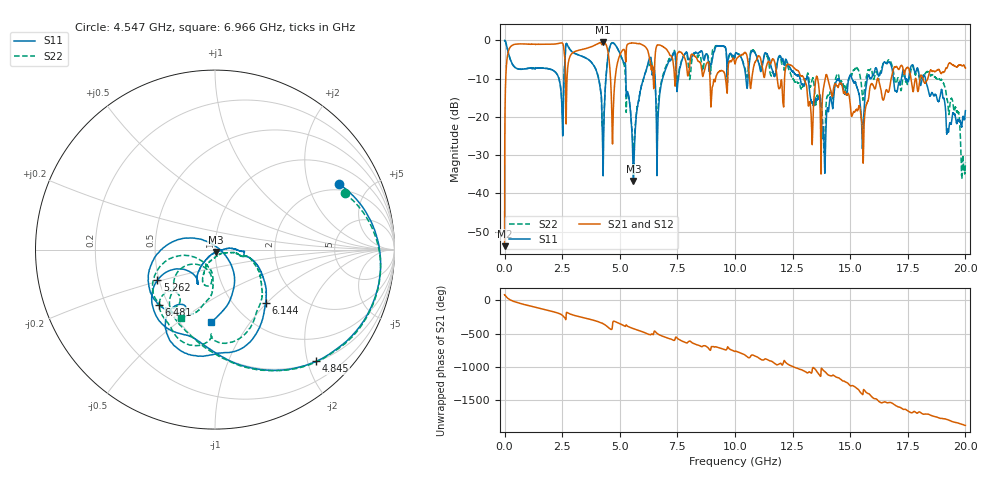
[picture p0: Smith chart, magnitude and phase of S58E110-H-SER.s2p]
!{S58E110}
!Johanson Technology Inc.
!www.johansontechnology.com
!Test Board Conditions:
!Substrate Type  RO4350B
!Substrate Thickness  60 mil
!Substrate Dk  3.66
!TL Type: GCPW
!TL Trace Width  115 mil
!TL Gap  52 mil
!Electrode orientation  Horizontal
!DUT TOPOLOGY	SERIES
!Mounting Pad LxW  55x428 mil
! Created Wed Apr 14 11:01:08 2021
# mhz S ma R 50
! 2 Port Network Data from SP1.SP block
! freq  magS11  angS11  magS21  angS21  magS12  angS12  magS22  angS22
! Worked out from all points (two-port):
!   20001 points, 300 kHz to 20 GHz, reference 50 ohm
!   highest |S21| = -0.36 dB at 4.27 GHz (marker M1); lowest = -53.8 dB at 300 kHz (marker M2)
!   |S21| within 3 dB of the highest: 143.1 MHz to 2.59 GHz (2.447 GHz wide, 179 % of centre); 2.931 GHz to 4.498 GHz (1.567 GHz wide, 42.2 % of centre)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
!   lowest |S11| = -36.7 dB at 5.59 GHz (marker M3), VSWR 1.03, Z = 50.4 - j1.39 ohm
!   |S11| at or under -10 dB: 5.266 GHz to 6.028 GHz (762.5 MHz wide, 13.5 % of centre); 13.17 GHz to 14.93 GHz (1.76 GHz wide, 12.5 % of centre); 18.27 GHz to end of sweep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
!   |S22| runs from -36.0 to 0.0 dB; largest |S21 - S12| = 0.01
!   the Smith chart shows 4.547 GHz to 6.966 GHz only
!   S11 on the Smith chart (normalised r, x): 4.547 GHz: 1.71, +3.20; 4.845 GHz: 0.51, -2.16; 5.262 GHz: 0.49, -0.19; 6.144 GHz: 1.38, -0.99; 6.481 GHz: 0.44, -0.34; 6.966 GHz: 0.70, -0.67
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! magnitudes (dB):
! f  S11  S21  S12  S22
! 300 kHz  0.0  -53.8  -54.0  -0.1
! 107.3 MHz  -1.8  -4.7  -4.7  -1.8
! 255.3 MHz  -5.1  -1.7  -1.7  -5.1
! 2.474 GHz  -15.7  -0.6  -0.6  -15.2
! 3.334 GHz  -4.1  -2.4  -2.4  -4.1
! 4.27 GHz  -34.1  -0.4  -0.4  -24.5
! 4.547 GHz  -2.1  -5.8  -5.8  -2.1
! 4.845 GHz  -1.5  -7.6  -7.6  -1.6
! 5.262 GHz  -8.8  -5.5  -5.5  -12.5
! 5.59 GHz  -36.7  -0.7  -0.7  -29.1
! 6.144 GHz  -7.7  -1.9  -1.9  -7.9
! 6.481 GHz  -7.1  -11.9  -11.9  -7.3
! 6.667 GHz  -19.3  -1.2  -1.2  -16.9
! 6.966 GHz  -7.9  -2.0  -2.0  -7.4
! 10 GHz  -4.1  -6.1  -6.2  -4.3
! 13.33 GHz  -16.2  -24.8  -24.7  -10.6
! 13.85 GHz  -25.0  -12.0  -11.9  -27.8
! 14.43 GHz  -10.2  -11.9  -11.9  -8.9
! 15.53 GHz  -28.0  -23.5  -23.5  -14.5
! 16.67 GHz  -5.6  -13.5  -13.5  -5.1
! 18.98 GHz  -13.1  -8.4  -8.4  -10.5
! 20 GHz  -18.4  -7.2  -7.1  -31.9
